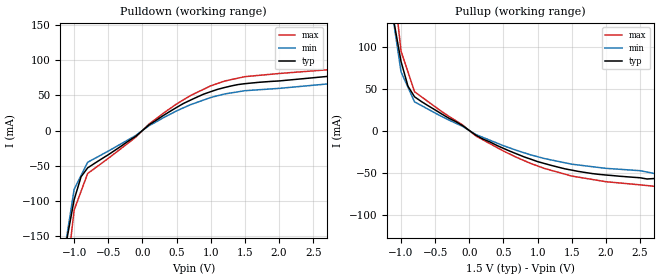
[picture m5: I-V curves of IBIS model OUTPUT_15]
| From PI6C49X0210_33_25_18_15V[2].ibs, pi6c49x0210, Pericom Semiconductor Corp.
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|   Model OUTPUT_15
[Model] OUTPUT_15
Model_type Output
Vref = 0.0000V
Rref = 500ohms
Vmeas = 0.750V
| variable   typ   min   max
C_comp   2.000pF   1.8pF	2.2pF
[Voltage Range]   1.5   1.425  1.575
[POWER Clamp Reference]   1.500V   NA   NA
[GND Clamp Reference]   0.000V   0	 0
[Pullup Reference]   1.5   1.425   1.575
[Pulldown Reference]   0.000V   NA   NA
[Temperature Range]   25.00   85.00   -45.000
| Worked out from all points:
|   slope of the pulldown table from 0 to 0.225 V, typ, clamps not added: 14.1 ohm
|   slope of the pullup table from 0 to 0.225 V, typ, clamps not added: 20.5 ohm
[Pulldown]
| Voltage   I(typ)   I(min)  I(max)
-2.501V   -1.346A    -1.144A    -1.548A
-1.1V     -151.1mA   NA         NA
-999.3mV  -97.83mA   -83.16mA   -112.5mA
-898.2mV  -65.44mA   NA         NA
-802mV    -52.94mA   -45mA      -60.88mA
-99.45mV  -8.35mA    -7.097mA   -9.602mA
301.5mV   21.02mA    17.87mA    24.17mA
999.4mV   55.02mA    46.77mA    63.27mA
1.5V      66.36mA    56.41mA    76.31mA
3.708V    85.7mA     74.84mA    93.55mA
3.801V    230.1mA    NA         NA
4.999V    1.25A      1.063A     1.438A
[Pullup]   |Note: Vtable = Vcc - Voutput
| Voltage   I(typ)   I(min)   I(max)
-2.501V   1.292A     1.098A     1.485A
-1.1V     128.3mA    NA         NA
-999.4mV  82.22mA    69.89mA    94.55mA
-898.2mV  52.83mA    NA         NA
-802mV    40.18mA    34.15mA    46.21mA
99.44mV   -5.76mA    -4.896mA   -6.624mA
898.2mV   -34.05mA   -28.94mA   -39.16mA
1.798V    -51.22mA   NA         NA
3.002V    -59.8mA    -55.83mA   -68.77mA
3.699V    -68.29mA   -65.3mA    -82.28mA
3.801V    -203.5mA   NA         NA
4.999V    -1.244A    -1.058A    -1.431A
[Ramp]
| variable   typ   min   max
dV/dt_r   2.0V/941.0p   2.0V/1041.0p   2.0V/841.0p
dV/dt_f   2.0V/806.0p   2.0V/1006.0p   2.0V/706.0p
R_load = 500ohms
